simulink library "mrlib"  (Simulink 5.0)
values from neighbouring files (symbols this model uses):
  fr0 = [phidr phiqr]    [imdef0vec.m]    (also in imdef1vec.m; imdefrotflux.m = sqrt(phidr^2+phiqr^2); imdefSIvec1.m)
  fs0 = fs    [calc0.m]    (also in imdef0vec.m = [phids phiqs]; imdef1vec.m = [phids phiqs]; imdefrotflux.m = [fs0d fs0q]; imdefSIvec1.m = [phids phiqs])
  ic = [fs0 fr0]    [imdef0vec.m]    (also in imdef1vec.m; imdef2vec.m = F; imic2.m = [phids phiqs phidr phiqr n0]'; imic3.m = [phids phiqs phidr phiqr n0]')
  Ra = .95    (= 0.95)    [altwdgs.m]    (also in Ccurverun.m = 0.018)
  wo = 2*pi*freq0    [calc0.m]    (also in IMabc2.m = 376.991118431; imabcparam.m = 376.991118431; IMabcrun0.m = 376.991118431; IMabcrun1.m = 376.991118431)
undefined symbols (not defined in the file or in its folder): fa0, fk0, L_1, phif0, Rf, Rkd, Rkq
libraries: simulink x3

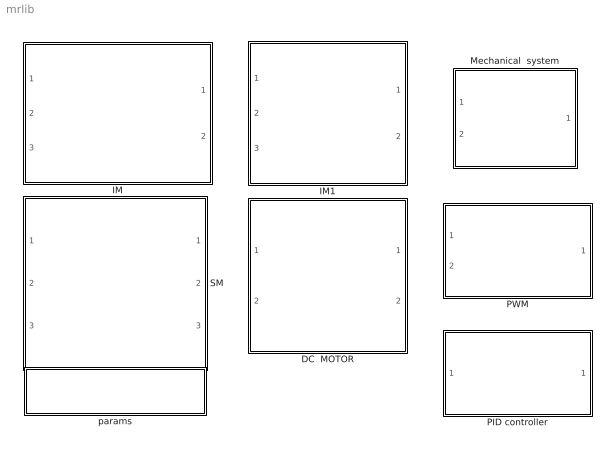
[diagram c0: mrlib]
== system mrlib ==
  DC  MOTOR : Subsystem  mask{Ra=2.0, La=5.2e-3, J=1.5e-4, Bm=1e-3, K=0.1}
      mask prompts: Ra "Armature resistance [ohm]"; La "Armature inductance [H]"; J "Moment of inertia [Kg.m^2]"; Bm "Frictional torque cefficient"; K "Electromechanical coupling coefficient [N.m/A]"
  IM : Subsystem  mask{Rs=0.02, Rr=0.01, Lsl=0.1, Lrl=0.1, Lm=5, wo=2*pi*60}
      mask prompts: Rs "Stator resistance [pu]"; Rr "Rotor resistance [pu]"; Lsl "Stator leakage inductance [pu]"; Lrl "Rotor leakage inductance [pu]"; Lm "Magnetizing inductance [pu]"; wo "Base frequency [rad/s]"
      mask help: Induction motor state space model in arbitrary reference frame. Parameters are expressed in per unit.
  IM1 : Subsystem  mask{Rs=0.5, Rr=0.5, Lsl=3e-3, Lrl=3e-3, Lm=100e-3, p=4, wo=2*pi*60}
      mask prompts: Rs "Stator resistance [Ohm]"; Rr "Rotor resistance [Ohm]"; Lsl "Stator leakage inductance [H]"; Lrl "Rotor leakage inductance [H]"; Lm "Magnetizing inductance [H]"; p "Number of poles"; wo "Base frequency [rad/s]"
  Mechanical  system : Subsystem  mask{H=0.3, B1=1e-5, B2=0, a=2}
      mask prompts: H "Inertia constant [s]"; B1 "Viscous damping coefficient"; B2 "Fan load factor"; a "Fan load exponent"
  PID controller : Subsystem  mask{Kp=1, Ki=10, Kd=0.1, sat=inf}
      mask prompts: Kp "Proportional gain (Kp)"; Ki "Integral gain (Ki)"; Kd "Derivative gain (Kd)"; sat "Saturation limit [pu]"
      mask help: Proportional-Integral Speed Controller
  PWM : Subsystem
  SM : Subsystem
  params : Subsystem

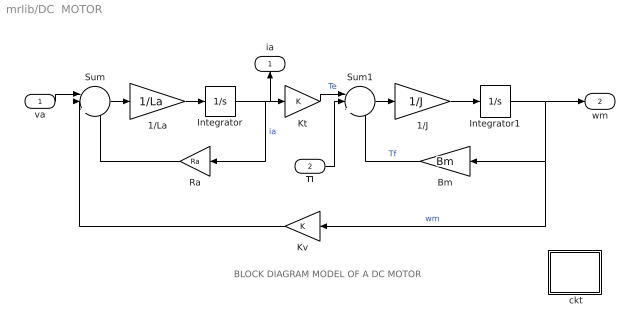
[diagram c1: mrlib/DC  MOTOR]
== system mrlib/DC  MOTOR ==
  note: BLOCK DIAGRAM MODEL OF A DC MOTOR
  va : Inport
  Tl : Inport  Port=2
  " ckt" : Subsystem
  1/J : Gain  Gain=1/J
  1/La : Gain  Gain=1/La
  Bm : Gain  Orientation=left  Gain=Bm
  Integrator : Integrator
  Integrator1 : Integrator
  Kt : Gain  Gain=K
  Kv : Gain  Orientation=left  Gain=K
  Ra : Gain  Orientation=left  Gain=Ra
  Sum : Sum  Inputs=||+--
  Sum1 : Sum  Inputs=||+--
  ia : Outport  Orientation=up
  wm : Outport  Port=2
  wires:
  Kv/1 -> Sum/2
  Ra/1 -> Sum/3
  Kt/1 -> Sum1/1  "Te"
  Bm/1 -> Sum1/3  "Tf"
  Sum/1 -> 1/La/1
  1/La/1 -> Integrator/1
  Integrator/1 -> Ra/1, Kt/1, ia/1  "ia"
  Sum1/1 -> 1/J/1
  1/J/1 -> Integrator1/1
  va/1 -> Sum/1
  Tl/1 -> Sum1/2
  Integrator1/1 -> Bm/1, Kv/1, wm/1  "wm"

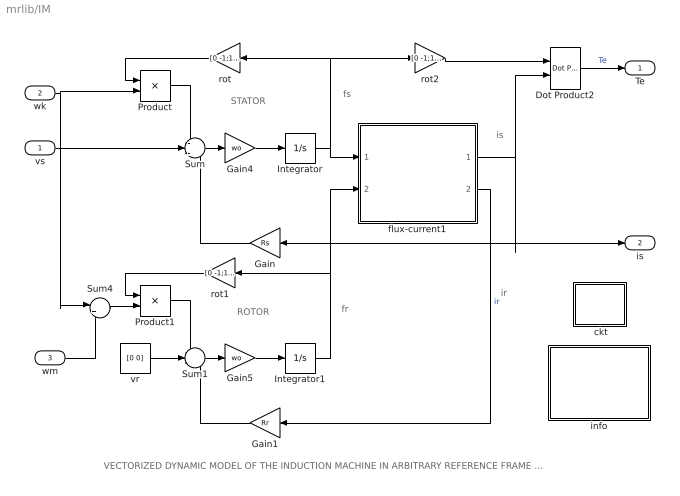
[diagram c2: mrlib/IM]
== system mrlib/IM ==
  note: ir
  note: VECTORIZED DYNAMIC MODEL OF THE INDUCTION MACHINE IN ARBITRARY REFERENCE FRAME (per unit formulation)
  note: is
  note: fr
  note: fs
  note: STATOR
  note: ROTOR
  vs : Inport
  wk : Inport  Port=2
  wm : Inport  Port=3
  " ckt" : Subsystem
  Dot Product2 : simulink/Math Operations/Dot Product
  Gain : Gain  Orientation=left  Gain=Rs
  Gain1 : Gain  Orientation=left  Gain=Rr
  Gain4 : Gain  Gain=wo
  Gain5 : Gain  Gain=wo
  Integrator : Integrator  InitialCondition=[ic(1) ic(2)]
  Integrator1 : Integrator  InitialCondition=[ic(3) ic(4)]
  Product : Product
  Product1 : Product
  Sum : Sum  Inputs=-+-
  Sum1 : Sum  Inputs=-+-
  Sum4 : Sum  Inputs=|+-
  flux-current1 : Subsystem
  info : Subsystem
  rot : Gain  Orientation=left  Gain=[0 -1;1 0]  Multiplication=Matrix(K*u)
  rot1 : Gain  Orientation=left  Gain=[0 -1;1 0]  Multiplication=Matrix(K*u)
  rot2 : Gain  Gain=[0 -1;1 0]  Multiplication=Matrix(K*u)
  vr : Constant  Value=[0 0]
  Te : Outport
  is : Outport  Port=2
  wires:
  wm/1 -> Sum4/2
  wk/1 -> Sum4/1, Product/2
  vs/1 -> Sum/2
  Dot Product2/1 -> Te/1  "Te"
  flux-current1/1(is) -> Dot Product2/2, is/1, Gain/1
  Gain5/1 -> Integrator1/1
  Sum1/1 -> Gain5/1
  Gain4/1 -> Integrator/1
  Sum/1 -> Gain4/1
  Sum4/1 -> Product1/2
  rot2/1 -> Dot Product2/1
  rot/1 -> Product/1
  Product/1 -> Sum/1
  rot1/1 -> Product1/1
  Product1/1 -> Sum1/1
  Integrator1/1 -> flux-current1/2(fr), rot1/1
  Integrator/1 -> rot2/1, rot/1, flux-current1/1(fs)
  flux-current1/2(ir) -> Gain1/1  "ir"
  Gain1/1 -> Sum1/3
  vr/1 -> Sum1/2
  Gain/1 -> Sum/3

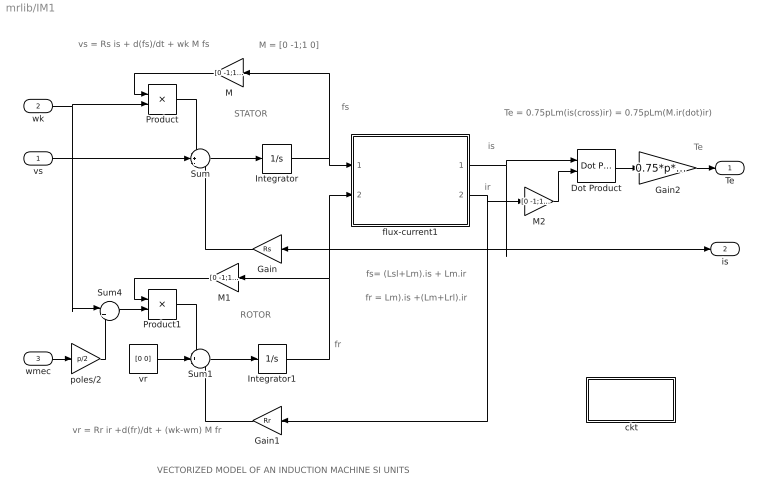
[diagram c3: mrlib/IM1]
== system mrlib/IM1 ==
  note: ROTOR
  note: STATOR
  note: fs
  note: is
  note: Te
  note: VECTORIZED MODEL OF AN INDUCTION MACHINE SI UNITS
  note: vs = Rs is + d(fs)/dt + wk M fs
  note: vr = Rr ir +d(fr)/dt + (wk-wm) M fr
  note: fs= (Lsl+Lm).is + Lm.ir
  note: fr = Lm).is +(Lm+Lrl).ir
  note: Te = 0.75pLm(is(cross)ir) = 0.75pLm(M.ir(dot)ir)
  note: M = [0 -1;1 0]
  note: ir
  note: fr
  vs : Inport
  wk : Inport  Port=2
  wmec : Inport  Port=3
  " ckt" : Subsystem
  Dot Product : simulink/Math Operations/Dot Product
  Gain : Gain  Orientation=left  Gain=Rs
  Gain1 : Gain  Orientation=left  Gain=Rr
  Gain2 : Gain  Gain=0.75*p*Lm
  Integrator : Integrator  InitialCondition=fs0
  Integrator1 : Integrator  InitialCondition=fr0
  M : Gain  Orientation=left  Gain=[0 -1;1 0]  Multiplication=Matrix(K*u)
  M1 : Gain  Orientation=left  Gain=[0 -1;1 0]  Multiplication=Matrix(K*u)
  M2 : Gain  Gain=[0 -1;1 0]  Multiplication=Matrix(K*u)
  Product : Product
  Product1 : Product
  Sum : Sum  Inputs=-+-
  Sum1 : Sum  Inputs=-+-
  Sum4 : Sum  Inputs=|+-
  flux-current1 : Subsystem
  poles/2 : Gain  Gain=p/2
  vr : Constant  Value=[0 0]
  Te : Outport
  is : Outport  Port=2
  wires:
  Gain/1 -> Sum/3
  vr/1 -> Sum1/2
  Gain1/1 -> Sum1/3
  Integrator/1 -> M/1, flux-current1/1(fs)
  Integrator1/1 -> flux-current1/2(fr), M1/1
  Product1/1 -> Sum1/1
  M1/1 -> Product1/1
  Product/1 -> Sum/1
  M/1 -> Product/1
  Sum4/1 -> Product1/2
  vs/1 -> Sum/2
  wk/1 -> Product/2, Sum4/1
  Sum1/1 -> Integrator1/1
  Sum/1 -> Integrator/1
  flux-current1/1(is) -> Gain/1, is/1, Dot Product/1
  Dot Product/1 -> Gain2/1
  Gain2/1 -> Te/1
  wmec/1 -> poles/2/1
  poles/2/1 -> Sum4/2
  M2/1 -> Dot Product/2
  flux-current1/2(ir) -> M2/1, Gain1/1

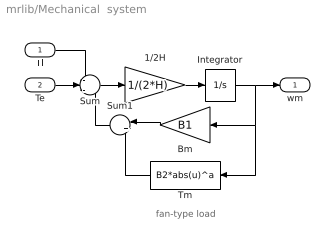
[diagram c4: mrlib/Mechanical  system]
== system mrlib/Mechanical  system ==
  note: fan-type load
  Tl : Inport
  Te : Inport  Port=2
  1/2H : Gain  Gain=1/(2*H)
  Bm : Gain  Orientation=left  Gain=B1
  Integrator : Integrator  InitialCondition=.82
  Sum : Sum  Inputs=-+-
  Sum1 : Sum  Orientation=left  Inputs=|++
  Tm : Fcn  Orientation=left  Expr=B2*abs(u)^a
  wm : Outport
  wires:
  Tl/1 -> Sum/1
  Te/1 -> Sum/2
  Integrator/1 -> wm/1, Bm/1, Tm/1
  Sum/1 -> 1/2H/1
  1/2H/1 -> Integrator/1
  Bm/1 -> Sum1/1
  Sum1/1 -> Sum/3
  Tm/1 -> Sum1/2

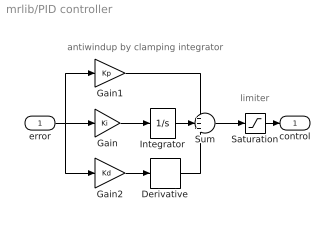
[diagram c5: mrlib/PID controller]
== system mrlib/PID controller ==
  note: antiwindup by clamping integrator
  note: limiter
  error : Inport
  Derivative : Derivative
  Gain : Gain  Gain=Ki
  Gain1 : Gain  Gain=Kp
  Gain2 : Gain  Gain=Kd
  Integrator : Integrator  LimitOutput=on  UpperSaturationLimit=sat  LowerSaturationLimit=-sat
  Saturation : Saturate  UpperLimit=sat  LowerLimit=-sat
  Sum : Sum  Inputs=+++
  control : Outport  InitialOutput=0
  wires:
  Gain1/1 -> Sum/1
  Gain/1 -> Integrator/1
  error/1 -> Gain/1, Gain1/1, Gain2/1
  Sum/1 -> Saturation/1
  Saturation/1 -> control/1
  Integrator/1 -> Sum/2
  Gain2/1 -> Derivative/1
  Derivative/1 -> Sum/3

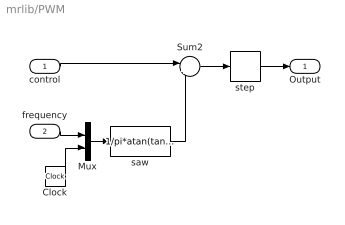
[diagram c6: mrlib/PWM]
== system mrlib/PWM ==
  control : Inport
  frequency : Inport  Port=2
  Clock : Clock
  Mux : Mux  Inputs=2
  Sum2 : Sum  Inputs=|+-
  saw : Fcn  Expr=1/pi*atan(tan((2*pi*u(1)*u(2)-pi)/2))+0.5
  step : Relay
  Output : Outport
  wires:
  Clock/1 -> Mux/2
  Mux/1 -> saw/1
  control/1 -> Sum2/1
  frequency/1 -> Mux/1
  saw/1 -> Sum2/2
  step/1 -> Output/1
  Sum2/1 -> step/1

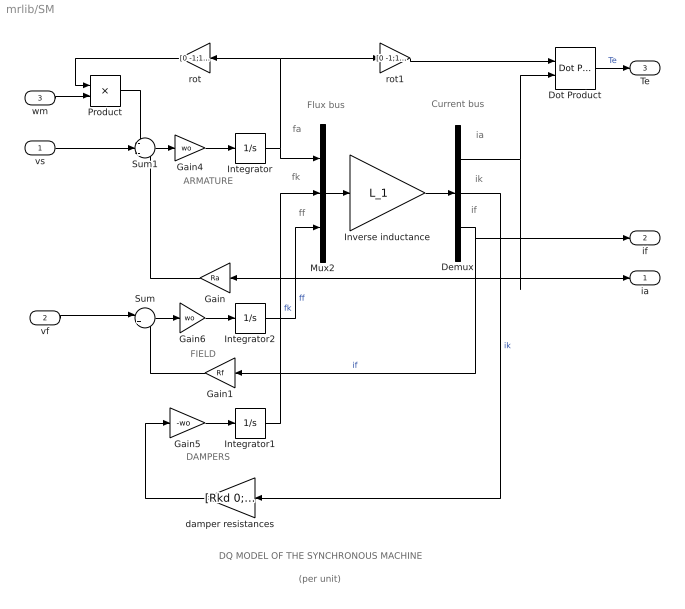
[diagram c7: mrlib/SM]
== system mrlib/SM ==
  note: DAMPERS
  note: ARMATURE
  note: fa
  note: ia
  note: FIELD
  note: DQ MODEL OF THE SYNCHRONOUS MACHINE
  note: Flux bus
  note: Current bus
  note: (per unit)
  note: fk
  note: ff
  note: ik
  note: if
  vs : Inport
  vf : Inport  Port=2
  wm : Inport  Port=3
  Demux : Demux  Outputs=3
  Dot Product : simulink/Math Operations/Dot Product
  Gain : Gain  Orientation=left  Gain=Ra
  Gain1 : Gain  Orientation=left  Gain=Rf
  Gain4 : Gain  Gain=wo
  Gain5 : Gain  Gain=-wo
  Gain6 : Gain  Gain=wo
  Integrator : Integrator  InitialCondition=fa0
  Integrator1 : Integrator  InitialCondition=fk0
  Integrator2 : Integrator  InitialCondition=phif0
  Inverse inductance : Gain  Gain=L_1  Multiplication=Matrix(K*u)
  Mux2 : Mux  Inputs=3
  Product : Product
  Sum : Sum  Inputs=|+-
  Sum1 : Sum  Inputs=-+-
  damper resistances : Gain  Orientation=left  Gain=[Rkd 0;0 Rkq]  Multiplication=Matrix(K*u)
  rot : Gain  Orientation=left  Gain=[0 -1;1 0]  Multiplication=Matrix(K*u)
  rot1 : Gain  Gain=[0 -1;1 0]  Multiplication=Matrix(K*u)
  ia : Outport
  if : Outport  Port=2
  Te : Outport  Port=3
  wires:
  Product/1 -> Sum1/1
  rot/1 -> Product/1
  wm/1 -> Product/2
  Gain5/1 -> Integrator1/1
  damper resistances/1 -> Gain5/1
  Integrator/1 -> Mux2/1, rot/1, rot1/1
  Sum1/1 -> Gain4/1
  Gain4/1 -> Integrator/1
  vs/1 -> Sum1/2
  Gain/1 -> Sum1/3
  Gain6/1 -> Integrator2/1
  Sum/1 -> Gain6/1
  vf/1 -> Sum/1
  Gain1/1 -> Sum/2
  rot1/1 -> Dot Product/1
  Demux/1 -> Gain/1, ia/1, Dot Product/2
  Dot Product/1 -> Te/1  "Te"
  Mux2/1 -> Inverse inductance/1
  Inverse inductance/1 -> Demux/1
  Integrator1/1 -> Mux2/2  "fk"
  Integrator2/1 -> Mux2/3  "ff"
  Demux/2 -> damper resistances/1  "ik"
  Demux/3 -> if/1, Gain1/1  "if"

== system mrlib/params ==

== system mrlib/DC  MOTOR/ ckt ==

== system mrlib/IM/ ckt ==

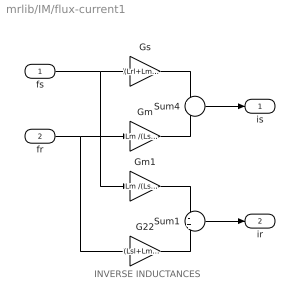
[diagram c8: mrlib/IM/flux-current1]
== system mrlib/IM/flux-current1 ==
  note: INVERSE INDUCTANCES
  fs : Inport
  fr : Inport  Port=2
  G22 : Gain  Gain=(Lsl+Lm )/(Lsl*Lrl+Lsl*Lm+Lrl*Lm)
  Gm : Gain  Gain=Lm /(Lsl*Lrl+Lsl*Lm+Lrl*Lm)
  Gm1 : Gain  Gain=Lm /(Lsl*Lrl+Lsl*Lm+Lrl*Lm)
  Gs : Gain  Gain=(Lrl+Lm) /(Lsl*Lrl+Lsl*Lm+Lrl*Lm)
  Sum1 : Sum  Inputs=-+
  Sum4 : Sum  Inputs=+-
  is : Outport
  ir : Outport  Port=2
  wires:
  Sum1/1 -> ir/1
  G22/1 -> Sum1/2
  Gm1/1 -> Sum1/1
  Sum4/1 -> is/1
  Gm/1 -> Sum4/2
  fr/1 -> G22/1, Gm/1
  Gs/1 -> Sum4/1
  fs/1 -> Gm1/1, Gs/1

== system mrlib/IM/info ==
  note: Electrical system equations: vs = Rs is + 1/wo (dfs/dt) + wk M(pi/2) fs vr = Rr ir + 1/wo (dfr/dt) + (wk - wm) M(pi/2) fr where the variables i, v, and f are 2-dimensional space vectors; for instance is = [ids iqs] and so forth, wk is the speed of the reference frame, wm the rotor speed, and M(pi/2)represents a 90o space rotator namely M(pi/2) = [0 -1;1 0] The flux linkage current relations are: fs = Ls is + Lm ir or is = Gs fs - Gm fr fr = Lm is + Lr ir ir = -Gm fs + Gr fr where Ls =Lm +Lsl and Lr = Lm +Lrl Gs = Lr / delta ; Gm = Lm / delta ; Gr= Ls / delta delta = Lsl*Lrl + Lm*Lsl + Lm* Lrl Mechanical system equations: Te = 2H (dwm/dt ) + Bm wm + Tl where Te = fs (cross) is = M(pi/2) fs (dot) is = fds iqs - fqs ids = fs x is = M(pi/2) fs . is = ir x fr = Lm (ir x is) = Lm/Lr (fr x is) = Gm (fr x fs)
  note: Mathematical model of the induction machine. Space vector formulation in an arbitrary dq common reference frame. Per unit description.

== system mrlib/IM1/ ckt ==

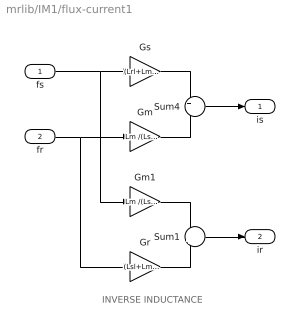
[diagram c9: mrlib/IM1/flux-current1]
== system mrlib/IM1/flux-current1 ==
  note: INVERSE INDUCTANCE
  fs : Inport
  fr : Inport  Port=2
  Gm : Gain  Gain=Lm /(Lsl*Lrl+Lsl*Lm+Lrl*Lm)
  Gm1 : Gain  Gain=Lm /(Lsl*Lrl+Lsl*Lm+Lrl*Lm)
  Gr : Gain  Gain=(Lsl+Lm )/(Lsl*Lrl+Lsl*Lm+Lrl*Lm)
  Gs : Gain  Gain=(Lrl+Lm) /(Lsl*Lrl+Lsl*Lm+Lrl*Lm)
  Sum1 : Sum  Inputs=-+
  Sum4 : Sum  Inputs=+-
  is : Outport
  ir : Outport  Port=2
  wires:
  fs/1 -> Gs/1, Gm1/1
  Gs/1 -> Sum4/1
  fr/1 -> Gm/1, Gr/1
  Gm/1 -> Sum4/2
  Sum4/1 -> is/1
  Gm1/1 -> Sum1/1
  Gr/1 -> Sum1/2
  Sum1/1 -> ir/1
